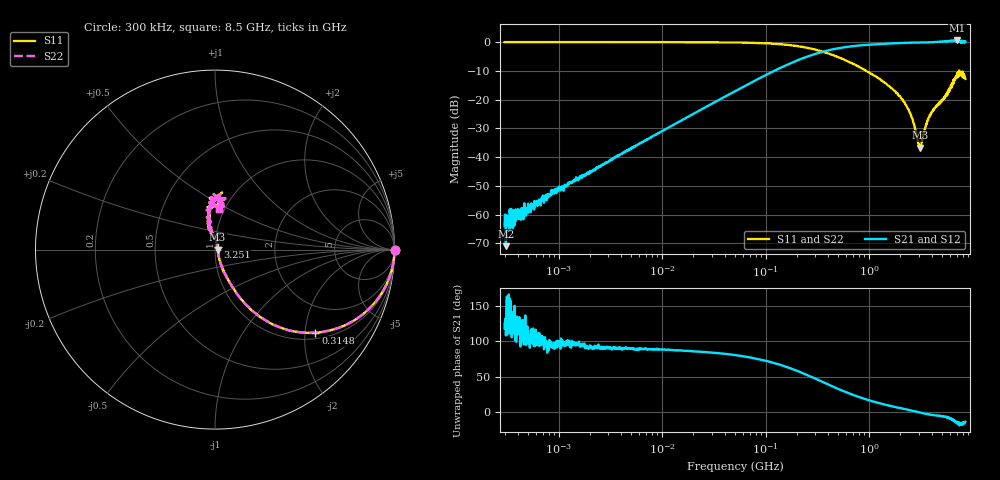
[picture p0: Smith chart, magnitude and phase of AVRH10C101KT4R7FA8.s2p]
! S-Parameter Data Generated by TDK Corporation
! Copyright(C) 2023 TDK Corporation.
! All Rights Reserved.
! TDK P/N: AVRH10C101KT4R7FA8 (Varistor)
! Property: V1mA=100V
! Size(LxWxT): 1x0.5x0.5mm
! Model Type: s2p (Touchstone File Format Version 1.0)
! Frequency: DC=Yes Start=0.3MHz Stop=8500MHz 1602points Log-sweep
! Model Generated on Oct. 12, 2023
! Port Assignments:
!  1 ---N--- 2
! Applicable Conditions:
!  Temperature = 25 degC
!  DC Bias Voltage = 0 V
!  Small Signal Operation
! Terms and conditions regarding TDK Simulation Models
! (1)This simulation model is being provided solely for informational purposes. Please refer to the specifications of the products in terms of detailed characteristics of such products.
! (2)In no event shall TDK Corporation of any of its subsidiaries be liable for any loss or damage arising, directly or indirectly,
!  From any information contained in this simulation model, including, but not limited to loss or damages arising from any inaccuracies, omissions or errors in connection with such information.
! (3)Any and all copyrights on this simulation model are owned by TDK Corporation.
!  Duplication or redistribution of this simulation model without prior written permission from TDK Corporation is prohibited.
! (4)This simulation model is subject to any modification or change without any prior notice.
! (5)Neither TDK Corporation nor any of its subsidiaries shall make any warranty, express or implied,
!  Including but not limited to the correctness, implied warranties of merchantability and fitness for a particular purpose with respect to this simulation models.
! (6)The use of this simulation model shall be deemed to have consented to the terms and conditions hereof.
# Hz S MA R 50
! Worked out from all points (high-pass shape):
!   1601 points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, 300 kHz to 8.5 GHz, reference 50 ohm
!   highest |S21| = 0.58 dB at 7.098 GHz (marker M1); lowest = -71.0 dB at 309 kHz (marker M2)
!   |S21| within 3 dB of the highest: 456.8 MHz to end of sweep
!   lowest |S11| = -36.7 dB at 3.072 GHz (marker M3), VSWR 1.03, Z = 51.5 + j0.00487 ohm
!   |S11| at or under -10 dB: 941.6 MHz to 7.422 GHz (6.48 GHz wide, 155 % of centre); 7.428 GHz to end of sweep
!   |S22| runs from -36.7 to 0.0 dB; largest |S21 - S12| = 0
!   S11 on the Smith chart (normalised r, x): 300 kHz: open; 314.8 MHz: 1.16, -2.27; 3.251 GHz: 1.03, +0.03; 8.5 GHz: 0.94, +0.45
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300000  1 -0.0  0.0006429 118.5  0.0006429 118.5  1 -0.0
309033  1 -0.0  0.0002827 108.4  0.0002827 108.4  1 -0.0
329356  1.001 -0.0  0.0007494 166.0  0.0007494 166.0  1.001 -0.0
363229  1.001 -0.0  0.0007825 138.2  0.0007825 138.2  1.001 -0.0
401618  1 -0.1  0.001244 110.1  0.001244 110.1  1 -0.1
1656733  1 -0.3  0.004549 95.7  0.004549 95.7  1 -0.3
9166247  0.9999 -1.5  0.02606 89.1  0.02606 89.1  0.9999 -1.5
5.049752e7  0.9872 -8.1  0.1401 80.8  0.1401 80.8  0.9872 -8.1
1.269478e8  0.9321 -19.3  0.3306 68.7  0.3306 68.7  0.9321 -19.3
2.806623e8  0.764 -36.7  0.5983 49.7  0.5983 49.7  0.764 -36.7
3.148314e8  0.7264 -39.6  0.6395 46.4  0.6395 46.4  0.7264 -39.6
6.59367e8  0.4419 -56.6  0.8421 26.0  0.8421 26.0  0.4419 -56.6
1.543407e9  0.1749 -66.2  0.943 9.8  0.943 9.8  0.1749 -66.2
2.294951e9  0.07765 -67.8  0.9733 4.2  0.9733 4.2  0.07765 -67.8
2.607409e9  0.04686 -62.1  0.9789 2.4  0.9789 2.4  0.04686 -62.1
3.07222e9  0.01468 0.2  0.9853 -0.0  0.9853 -0.0  0.01468 0.2
3.250993e9  0.02006 44.7  0.9858 -0.8  0.9858 -0.8  0.02006 44.7
3.912229e9  0.0537 83.3  0.9952 -3.1  0.9952 -3.1  0.0537 83.3
5.627128e9  0.1273 105.6  1.041 -6.8  1.041 -6.8  0.1273 105.6
7.097747e9  0.29 95.9  1.069 -15.7  1.069 -15.7  0.29 95.9
7.798873e9  0.2797 88.0  1.029 -15.8  1.029 -15.8  0.2797 88.0
8.5e9  0.2294 84.9  1.006 -13.1  1.006 -13.1  0.2294 84.9
